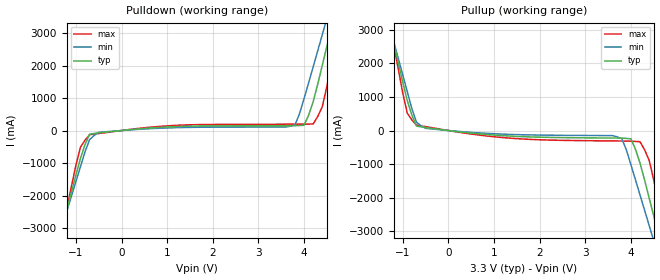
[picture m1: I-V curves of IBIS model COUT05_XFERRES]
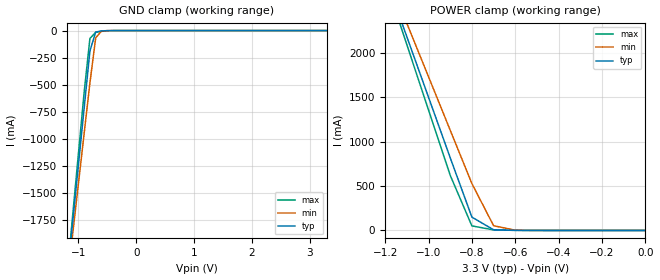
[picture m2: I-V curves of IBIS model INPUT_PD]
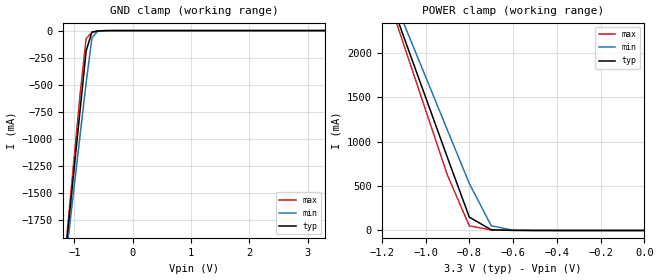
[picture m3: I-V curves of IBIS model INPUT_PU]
|   This file is an IBIS representation of the   |
|   Integrated Circuit Systems, Inc.   |
|   ICS83947I   |
[IBIS Ver]   3.2
[File name]   83947i.ibs
[File Rev]   1.0
[Date]   July 26 2002 | Last modified
|   July 26 2002 | Generated
[Source] Originated at Integrated Circuit Systems, Inc.
[Disclaimer]
(C) Copyright Integrated Circuit Systems, Inc. 1997
   All rights reserved
ICS hereby grants the user of this IBIS model a non-exclusive,
nontransferable license to use this IBIS model under the following terms.
Before using this IBIS model, the user should read this license.
If the user does not accept these terms,  the IBIS model should be
returned to ICS within 30 days.
   The user is granted this license only to use the IBIS model and
is not granted rights to sell, load, rent, lease or license the IBIS
model in whole or in part, or in modified form to anyone other than
user. User may modify the IBIS model to suit its specific
applications but rights to derivative works and such modifications
shall belong to ICS.
   This IBIS model is provided on an "AS IS" basis and ICS makes
absolutely no warranty with respect to the information contained
herein. ICS DISCLAIMS AND CUSTOMER WAIVES ALL WARRANTIES, EXPRESS
OR IMPLIED, INCLUDING WARRANTIES OF MERCHANTABILITY OR FITNESS FOR
A PARTICULAR PURPOSE. The entire risk as to quality and performance
is with the Customer. ACCORDINGLY, IN NO EVENT SHALL THE COMPANY BE
LIABLE FOR ANY DAMAGES, WHETHER IN CONTRACT OR TORT,INCLUDING ANY
LOST PROFITS OR OTHER INCIDENTAL, CONSEQUENTIAL, EXEMPLARY, OR
PUNITIVE DAMAGES ARISING OUT OF THE USE OR APPLICATION OF THE IBIS
model provided in this package. Further, ICS reserves the right to
make changes without notice to any product herein to improve
reliability, function, or design. ICS does not convey any license
under patent rights or any other intellectual property rights,
including those of third parties.
   ICS is not obligated to provide maintenance or support
for the licensed IBIS model.
[Copyright]   Copyright 2002 by Integrated Circuit Systems, Inc.
[Component]   ICS83947I
[Manufacturer] Integrated Circuit Systems, Inc.
[Package]
|   typ   min   max
R_pkg   8.5m   7.8m   9.2m
L_pkg   0.85nH   0.799nH   0.904nH
C_pkg   0.206pF   0.202pF   0.211pF
[Pin] signal_name   model_name
1   GND   GND
2   CLK_SEL   INPUT_PU
3   CLK0   INPUT_PU
4   CLK1   INPUT_PU
5   CLK_EN   INPUT_PU
6   OE   INPUT_PU
7   VDD   POWER
8   GND   GND
9   GND   GND
10   VDDO   POWER
11   Q8   COUT05_XFERRES
12   GND   GND
13   Q7   COUT05_XFERRES
14   VDDO   POWER
15   Q6   COUT05_XFERRES
16   GND   GND
17   GND   GND
18   VDDO   POWER
19   Q5   COUT05_XFERRES
20   GND   GND
21   Q4   COUT05_XFERRES
22   VDDO   POWER
23   Q3   COUT05_XFERRES
24   GND   GND
25   GND   GND
26   Q2   COUT05_XFERRES
27   VDDO   POWER
28   Q1   COUT05_XFERRES
29   GND   GND
30   Q0   COUT05_XFERRES
31   VDDO   POWER
32   GND   GND
| Models and submodels in the file (3): COUT05_XFERRES (Output), INPUT_PD (Input), INPUT_PU (Input)
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|   ICS83947I 3.3V Clock Drive Model
| This model is suitable for all output pins on the
|  ICS83947I
[Model]   COUT05_XFERRES
Model_type   Output
Polarity   Non-Inverting
|   typ   min   max
C_comp   2pF   1.5pF   2.5pF
|   typ   min   max
[Voltage range]  3.3V   3.15V   3.45V
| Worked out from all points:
|   slope of the pulldown table from 0 to 0.495 V, typ, clamps not added: 7.71 ohm
|   slope of the pullup table from 0 to 0.495 V, typ, clamps not added: 6.44 ohm
[pulldown]
|Voltage   I (typ)   I (min)   I (max)
-3.3V     -13.74A    -12.12A    -16.25A
-1.4V     -3.526A    -3.407A    -3.72A
-1.3V     -2.987A    -2.948A    -3.058A
-900mV    -857.7mA   -1.112A    -513.9mA
-700mV    -114.2mA   -281.1mA   -130.4mA
3.8V      149.8mA    170.1mA    194.9mA
4V        161.9mA    982.2mA    196.3mA
4.2V      887.5mA    1.963A     202.2mA
4.4V      2.009A     2.952A     734.1mA
4.6V      3.173A     3.944A     2.074A
4.8V      4.339A     4.937A     3.509A
6.6V      15.05A     14.04A     16.69A
[pullup]
|Voltage   I (typ)   I (min)   I (max)
-3.3V     15.02A     13.23A     17.78A
-1.3V     3.212A     3.164A     3.296A
-900mV    885.7mA    1.151A     514.2mA
-700mV    133mA      248.7mA    161.5mA
3.6V      -223.7mA   -151.5mA   -310mA
3.8V      -226.2mA   -242.1mA   -312.1mA
4V        -247.6mA   -1.022A    -317.2mA
4.3V      -1.48A     -2.38A     -576.5mA
4.5V      -2.547A    -3.289A    -1.474A
4.6V      -3.081A    -3.743A    -2.13A
4.8V      -4.149A    -4.654A    -3.444A
6.6V      -13.78A    -12.87A    -15.26A
[Ramp]
|   typ   min   max
dV/dt_r   1.98/0.6n   1.98/0.80n   1.98/0.4n
dV/dt_f   1.98/0.6n   1.98/0.80n   1.98/0.4n
[Model]   INPUT_PD
Model_type   Input
Polarity   Non-Inverting
Vinl = 1.4V
Vinh = 1.85V
|   typ   min   max
C_comp   2pF   1.5pF   2.5pF
|   typ   min   max
[Voltage range]  3.3V   3.15V   3.45V
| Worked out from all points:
|   GND clamp passes 1 mA (typ) near -0.51 V on its own axis
|   POWER clamp passes 1 mA (typ) near -0.60 V on its own axis
[GND_clamp]
|Voltage I(typ)   I(min)   I(max)
-3.3V     -13.52A    -12.28A    -14.38A
-1.2V     -2.314A    -2.362A    -2.296A
-1.1V     -1.782A    -1.891A    -1.721A
-1V       -1.25A     -1.422A    -1.146A
-900mV    -718.5mA   -952.6mA   -572.1mA
-800mV    -188.2mA   -484.5mA   -72.95mA
-700mV    -13.66mA   -66.68mA   -15.82mA
-600mV    -3.044mA   -4.415mA   -6.968mA
-500mV    -658.9uA   -400.5uA   -2.169mA
3.3V      64.58uA    64.62uA    64.6uA
[POWER_clamp]
|Voltage   I(typ)   I(min)   I(max)
-3.3V     17.27A     15.67A     18.38A
-1.2V     2.866A     2.938A     2.832A
-1.1V     2.183A     2.334A     2.094A
-1V       1.501A     1.732A     1.358A
-900mV    819.8mA    1.13A      621.9mA
-800mV    150.3mA    528.4mA    51.58mA
-700mV    7.809mA    53.45mA    6.607mA
-600mV    968.4uA    3.161mA    1.955mA
0V        64.58uA    61.35uA    67.83uA
[Model]   INPUT_PU
Model_type   Input
Polarity   Non-Inverting
Vinl = 1.4V
Vinh = 1.85V
|   typ   min   max
C_comp   2pF   1.5pF   2.5pF
|   typ   min   max
[Voltage range]  3.3V   3.15V   3.45V
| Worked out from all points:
|   GND clamp passes 1 mA (typ) near -0.51 V on its own axis
|   POWER clamp passes 1 mA (typ) near -0.60 V on its own axis
[GND_clamp]
|Voltage   I(typ)   I(min)   I(max)
-3.3V     -13.52A    -12.28A    -14.38A
-1.2V     -2.314A    -2.362A    -2.296A
-1.1V     -1.782A    -1.891A    -1.721A
-1V       -1.25A     -1.422A    -1.146A
-900mV    -718.6mA   -952.7mA   -572.2mA
-800mV    -188.2mA   -484.6mA   -73.02mA
-700mV    -13.72mA   -66.74mA   -15.89mA
-600mV    -3.109mA   -4.477mA   -7.036mA
-500mV    -723.5uA   -462.1uA   -2.236mA
3.3V      3.748nA    2.972uA    -2.918uA
[POWER_clamp]
|Voltage   I(typ)   I(min)   I(max)
-3.3V     17.27A     15.67A     18.38A
-1.2V     2.866A     2.938A     2.832A
-1.1V     2.183A     2.334A     2.094A
-1V       1.501A     1.732A     1.358A
-900mV    819.7mA    1.129A     621.8mA
-800mV    150.2mA    528.4mA    51.51mA
-700mV    7.744mA    53.39mA    6.54mA
-600mV    903.9uA    3.099mA    1.887mA
0V        3.748nA    2.31nA     19.96nA
